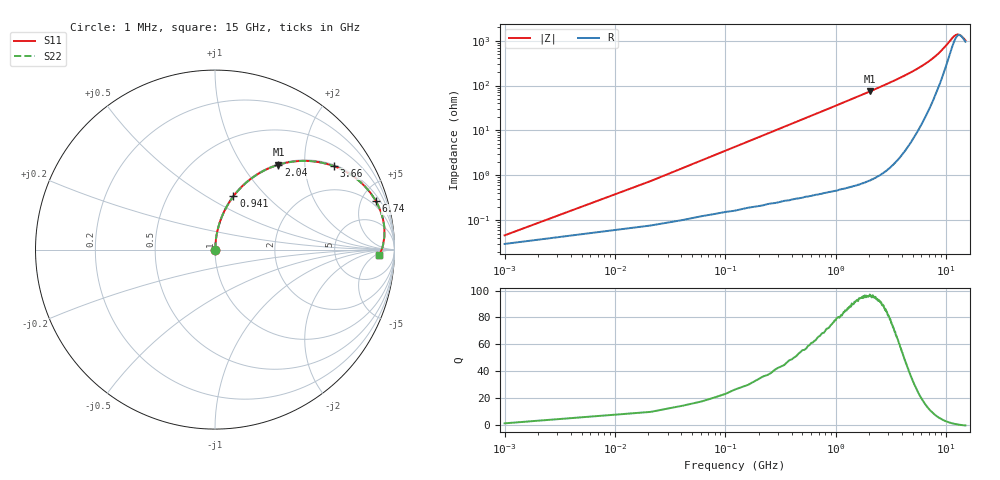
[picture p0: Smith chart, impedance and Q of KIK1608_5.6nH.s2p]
!version-2
!date-01.2022
!Series
# MHz S RI R 50
!Freq ReS11 ImS11 ReS21 ImS21 ReS12 ImS12 ReS22 ImS22
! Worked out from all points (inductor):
!   751 points, 1 MHz to 15 GHz, reference 50 ohm
!   read as one part in series: L = 5.6 nH near 61 MHz
!   highest Q = 95.9 at 2.04 GHz (marker M1), where L = 5.75 nH
!   self-resonance near 13.57 GHz
!   S11 on the Smith chart (normalised r, x): 1 MHz: 1.00, +0.00; 941 MHz: 1.01, +0.67; 2.04 GHz: 1.02, +1.47; 3.66 GHz: 1.04, +2.80; 6.74 GHz: 1.48, +6.47; 15 GHz: 20, -7
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1  0.000293 0.000352  0.9997 -0.000352  0.9997 -0.000352  0.000293 0.000352
41  0.00123 0.0144  0.9988 -0.0144  0.9988 -0.0144  0.00123 0.0144
81  0.00218 0.0284  0.9978 -0.0284  0.9978 -0.0284  0.00218 0.0284
121  0.00345 0.0424  0.9966 -0.0424  0.9966 -0.0424  0.00345 0.0424
161  0.00505 0.0563  0.9949 -0.0563  0.9949 -0.0563  0.00505 0.0563
201  0.00702 0.0701  0.993 -0.0701  0.993 -0.0701  0.00702 0.0701
321  0.0151 0.111  0.9849 -0.111  0.9849 -0.111  0.0151 0.111
481  0.0308 0.1638  0.9692 -0.1638  0.9692 -0.1638  0.0308 0.1638
681  0.0577 0.2256  0.9423 -0.2256  0.9423 -0.2256  0.0577 0.2256
941  0.1029 0.2973  0.8971 -0.2973  0.8971 -0.2973  0.1029 0.2973
1420  0.2067 0.3994  0.7933 -0.3994  0.7933 -0.3994  0.2067 0.3994
2040  0.3534 0.4729  0.6466 -0.4729  0.6466 -0.4729  0.3534 0.4729
2520  0.4604 0.493  0.5396 -0.493  0.5396 -0.493  0.4604 0.493
3660  0.6606 0.4657  0.3394 -0.4657  0.3394 -0.4657  0.6606 0.4657
5020  0.8054 0.3808  0.1946 -0.3808  0.1946 -0.3808  0.8054 0.3808
6740  0.8968 0.2697  0.1032 -0.2697  0.1032 -0.2697  0.8968 0.2697
7520  0.9184 0.2249  0.0816 -0.2249  0.0816 -0.2249  0.9184 0.2249
10020  0.9443 0.1087  0.0556 -0.1087  0.0556 -0.1087  0.9443 0.1087
11560  0.9419 0.0548  0.0581 -0.0548  0.0581 -0.0548  0.9419 0.0548
12520  0.9365 0.0267  0.0635 -0.0267  0.0635 -0.0267  0.9365 0.0267
13480  0.9292 0.00218  0.0708 -0.00218  0.0708 -0.00218  0.9292 0.00218
15000  0.9151 -0.0302  0.0848 0.0302  0.0848 0.0302  0.9151 -0.0302
